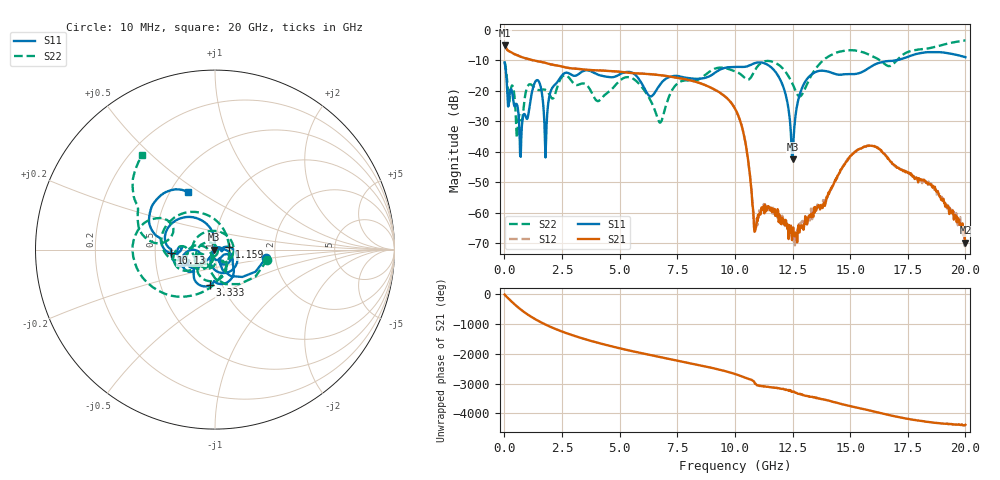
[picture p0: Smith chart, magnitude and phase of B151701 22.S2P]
!  2-Port S-parameters saved by WinCal
! VAR MeasName=S-Parameters (CALIBRATED_DATA) read from VNA (N5244A)
! VAR MeasDate=2015-12-24 19:10:42
! VAR NAME=B151701 22
! VAR FILENAME=B151701 22.S2P
! VAR DATE=2015-12-24 19:10:42
! VAR PHYS_PORTS=1,3
# Hz S DB R 50
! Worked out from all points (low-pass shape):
!   801 points, 10 MHz to 20 GHz, reference 50 ohm
!   highest |S21| = -5.13 dB at 10 MHz (marker M1); lowest = -69.9 dB at 20 GHz (marker M2)
!   |S21| within 3 dB of the highest: start of sweep to 459.9 MHz
!   lowest |S11| = -42.5 dB at 12.5 GHz (marker M3), VSWR 1.02, Z = 49.3 - j0.0508 ohm
!   |S11| at or under -10 dB: start of sweep to 17.06 GHz
!   |S22| runs from -35.5 to -3.6 dB; largest |S21 - S12| = 0.0015
!   S11 on the Smith chart (normalised r, x): 10 MHz: 1.79, -0.18; 1.159 GHz: 1.17, +0.03; 3.333 GHz: 0.88, -0.36; 10.13 GHz: 0.61, -0.02; 20 GHz: 0.61, +0.45
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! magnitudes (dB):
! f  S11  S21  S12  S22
! 10 MHz  -10.8  -5.1  -5.1  -10.5
! 609.7 MHz  -27.6  -8.6  -8.6  -29.4
! 1.159 GHz  -22.0  -9.9  -9.9  -18.0
! 1.484 GHz  -16.9  -10.4  -10.4  -19.8
! 1.809 GHz  -35.7  -11.0  -11.0  -19.9
! 2.109 GHz  -18.8  -11.6  -11.6  -22.6
! 3.333 GHz  -14.0  -13.0  -13.0  -17.7
! 3.358 GHz  -13.8  -13.0  -13.0  -17.7
! 5.532 GHz  -14.1  -14.2  -14.2  -15.9
! 6.682 GHz  -18.8  -14.9  -14.9  -29.7
! 7.581 GHz  -15.3  -15.9  -15.9  -17.3
! 10.01 GHz  -12.2  -25.9  -25.9  -13.7
! 10.13 GHz  -12.2  -27.9  -27.9  -14.1
! 10.5 GHz  -12.1  -39.1  -39.2  -16.3
! 10.88 GHz  -11.0  -65.9  -65.0  -13.2
! 11.95 GHz  -16.2  -62.7  -61.4  -11.9
! 12.5 GHz  -42.5  -67.2  -68.6  -17.8
! 12.83 GHz  -20.9  -65.1  -63.5  -21.9
! 13.35 GHz  -14.6  -60.7  -62.1  -14.5
! 15.25 GHz  -14.5  -40.0  -40.0  -6.9
! 16.68 GHz  -10.3  -42.6  -42.5  -12.0
! 20 GHz  -9.1  -69.9  -66.2  -3.6
